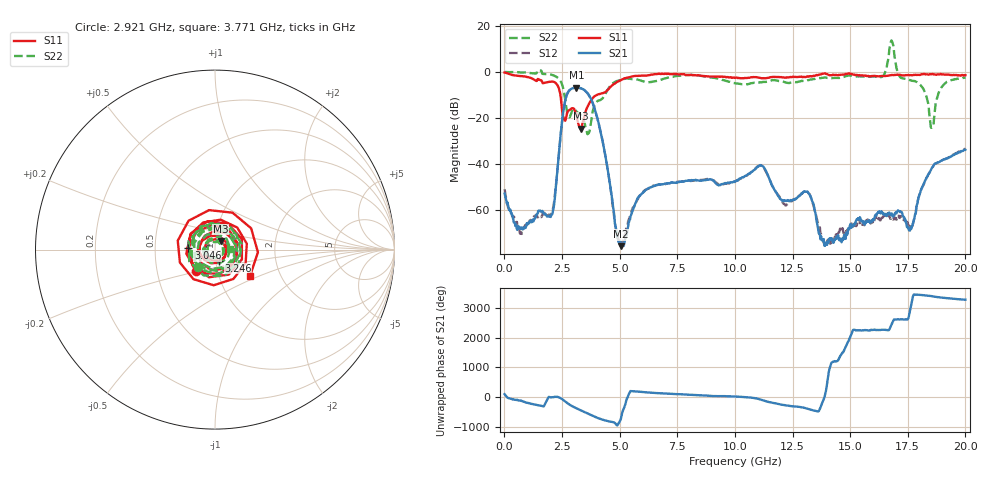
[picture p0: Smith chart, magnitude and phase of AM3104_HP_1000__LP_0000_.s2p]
!Created with skrf (http://scikit-rf.org).
# Hz S RI R 50.0
!freq ReS11 ImS11 ReS21 ImS21 ReS12 ImS12 ReS22 ImS22
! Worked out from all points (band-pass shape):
!   1601 points, 10 MHz to 20 GHz, reference 50 ohm
!   highest |S21| = -6.80 dB at 3.121 GHz (marker M1); lowest = -75.8 dB at 5.045 GHz (marker M2)
!   |S21| within 3 dB of the highest: 2.716 GHz to 3.647 GHz (930.5 MHz wide, 29.2 % of centre)
!   lowest |S11| = -24.7 dB at 3.333 GHz (marker M3), VSWR 1.12, Z = 53.2 + j5.08 ohm
!   |S11| at or under -10 dB: 2.43 GHz to 4.025 GHz (1.595 GHz wide, 49.4 % of centre)
!   |S22| runs from -27.1 to 13.7 dB; largest |S21 - S12| = 0.025
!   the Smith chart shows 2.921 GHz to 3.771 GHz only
!   S11 on the Smith chart (normalised r, x): 2.921 GHz: 0.79, -0.20; 3.046 GHz: 0.74, +0.01; 3.246 GHz: 1.03, -0.13; 3.771 GHz: 1.40, -0.44
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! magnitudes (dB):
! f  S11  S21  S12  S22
! 10 MHz  -0.3  -53.0  -51.0  -0.1
! 672.2 MHz  -1.8  -68.3  -70.3  -0.2
! 2.021 GHz  -4.2  -62.7  -62.0  -1.2
! 2.584 GHz  -20.5  -15.5  -15.5  -8.6
! 2.921 GHz  -15.9  -7.3  -7.4  -17.3
! 3.046 GHz  -16.6  -7.0  -7.0  -16.2
! 3.121 GHz  -18.3  -6.8  -6.8  -17.2
! 3.246 GHz  -23.8  -6.9  -7.0  -18.4
! 3.333 GHz  -24.7  -7.2  -7.2  -18.9
! 3.346 GHz  -24.6  -7.2  -7.3  -19.1
! 3.771 GHz  -12.2  -12.0  -12.1  -21.4
! 5.045 GHz  -3.6  -75.8  -74.1  -3.6
! 6.682 GHz  -0.9  -49.0  -49.2  -3.7
! 10.01 GHz  -2.6  -47.9  -47.7  -4.9
! 11.14 GHz  -2.7  -40.8  -40.7  -4.5
! 13.34 GHz  -2.0  -56.1  -55.8  -3.3
! 13.97 GHz  -0.9  -74.3  -75.0  -2.6
! 16.68 GHz  -1.5  -61.9  -62.7  7.2
! 17.61 GHz  -1.4  -68.1  -67.3  -3.6
! 18.54 GHz  -0.9  -41.9  -42.0  -24.3
! 19 GHz  -1.1  -38.5  -38.4  -6.2
! 20 GHz  -1.4  -33.9  -33.5  -2.5
